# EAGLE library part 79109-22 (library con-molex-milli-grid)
RECEPTACAL
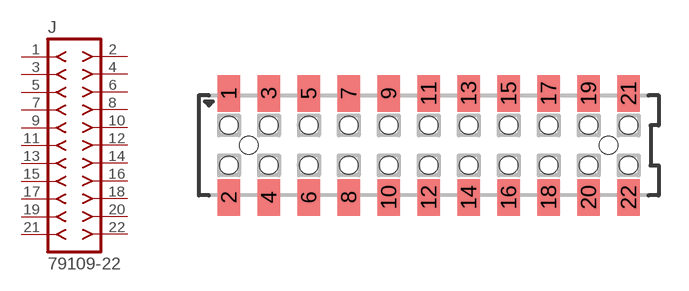
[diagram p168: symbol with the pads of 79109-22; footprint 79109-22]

Designator prefix J

## 79109-22  [79109-22]
1  1  pas
2  2  pas
3  3  pas
4  4  pas
5  5  pas
6  6  pas
7  7  pas
8  8  pas
9  9  pas
10  10  pas
11  11  pas
12  12  pas
13  13  pas
14  14  pas
15  15  pas
16  16  pas
17  17  pas
18  18  pas
19  19  pas
20  20  pas
21  21  pas
22  22  pas

## Footprint 79109-22 (pad centres in mm)
RECEPTACAL SMD Dual Row, Vertical, Pass-Thru
smd 1.12 x 1.83: 1 -10,2.6; 2 -10,-2.6; 3 -8,2.6; 4 -8,-2.6; 5 -6,2.6; 6 -6,-2.6; 7 -4,2.6; 8 -4,-2.6; 9 -2,2.6; 10 -2,-2.6; 11 0,2.6; 12 0,-2.6; 13 2,2.6; 14 2,-2.6; 15 4,2.6; 16 4,-2.6; 17 6,2.6; 18 6,-2.6; 19 8,2.6; 20 8,-2.6; 21 10,2.6; 22 10,-2.6
hole 0.914 at -9,0
hole 0.914 at -10,1
hole 0.914 at -10,-1
hole 0.914 at -8,-1
hole 0.914 at -8,1
hole 0.914 at -6,-1
hole 0.914 at -6,1
hole 0.914 at 9,0
hole 0.914 at -4,1
hole 0.914 at -4,-1
hole 0.914 at -2,1
hole 0.914 at -2,-1
hole 0.914 at 0,1
hole 0.914 at 0,-1
hole 0.914 at 2,1
hole 0.914 at 2,-1
hole 0.914 at 4,-1
hole 0.914 at 4,1
hole 0.914 at 6,1
hole 0.914 at 6,-1
hole 0.914 at 8,1
hole 0.914 at 8,-1
hole 0.914 at 10,1
hole 0.914 at 10,-1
